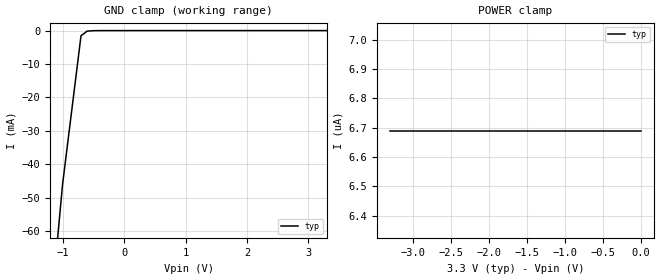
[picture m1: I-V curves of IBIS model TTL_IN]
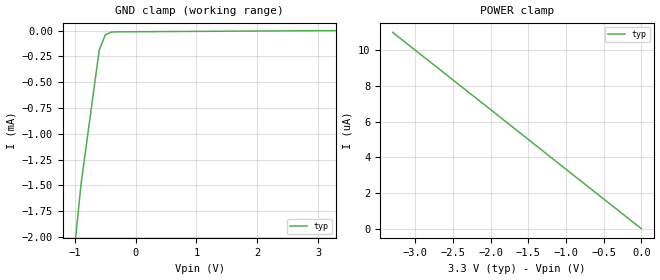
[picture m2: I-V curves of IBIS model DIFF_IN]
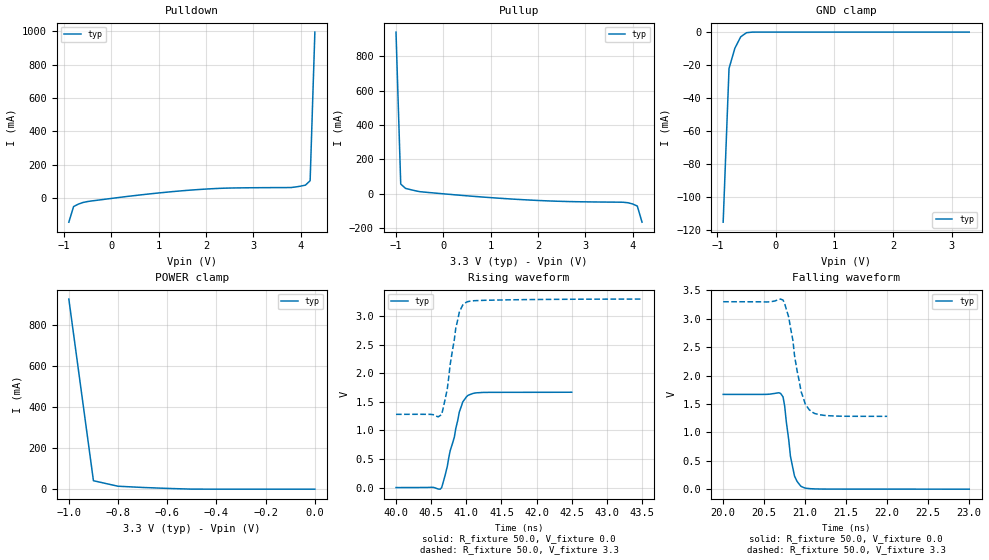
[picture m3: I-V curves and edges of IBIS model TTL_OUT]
|   Texas Instruments Incorporated
|   Data Transmissions Products
|   IBIS Model for SN65LVDS152
|   32DA Package
[IBIS Ver]   3.2
[Comment char]   |_char
[File name]   lvds152.ibs
[File Rev]   1.0
[Date]   11Dec00
[Source]   File originated at Texas Instruments Incorporated.
   Data Transmission Products Group. All data based on
   Bench Measurements.
[Notes]   File created by Thomas Fisher
[Disclaimer]
(C) Copyright Texas Instruments Incorporated 2000
   All rights reserved
  Texas Instruments Incorporated hereby grants the user of this IBIS
model a non-exclusive, nontransferable license to use this IBIS model
under the following terms.  Before using this IBIS model, the user
should read this license.  If the user does not accept these terms,
the IBIS model should be returned to Texas Instruments within 30 days.
  The user is granted this license only to use the IBIS model and
is not granted rights to sell, load, rent, lease or license the IBIS
model in whole or in part, or in modified form to anyone other than
user.  User may modify the IBIS model to suit its specific applications
but rights to derivative works and such modifications shall belong to
Texas Instruments.
  This IBIS model is provided on an "AS IS" basis and Texas Instruments
makes absolutely no warranty with respect to the information contained
herein.  TEXAS INSTRUMENTS DISCLAIMS AND CUSTOMER WAIVES ALL WARRANTIES,
EXPRESS OR IMPLIED, INCLUDING WARRANTIES OF MERCHANTABILITY OR FITNESS
FOR A PARTICULAR PURPOSE. The entire risk as to quality and performance
is with the Customer. ACCORDINGLY, IN NO EVENT SHALL THE COMPANY BE LIABLE
FOR ANY DAMAGES, WHETHER IN CONTRACT OR TORT,INCLUDING ANY LOST PROFITS
OR OTHER INCIDENTAL, CONSEQUENTIAL, EXEMPLARY, OR PUNITIVE DAMAGES ARISING
OUT OF THE USE OR APPLICATION OF THE IBIS model provided in this package.
Further, Texas Instruments reserves the right to discontinue or make changes
without notice to any product herein to improve reliability, function, or
design. Texas Instruments does not convey any license under patent rights
or any other intellectual property rights, including those of third parties.
Contact Texas Instruments at ATTN:DATA TRANSMISSIONS
[Copyright]   Copyright 2000, Texas Instruments, All Rights Reserved
[Component]   SN65LVDS152DA
[Manufacturer]  Texas Instruments Incorporated
[Package]
|   typ   min   max
R_pkg   0.002   0.001   0.003
L_pkg   1.466nH   1.067nH   2.360nH
C_pkg   0.459pF   0.360pF   0.629pF
[Pin] signal_name  model_name   R_pin   L_pin   C_pin
 1   DI+   DIFF_IN   0.003   2.347n   0.610p
 2   DI-   DIFF_IN   0.002   1.869n   0.531p
 3   GND   GND   0.001   1.487n   0.496p
 4   LCI+   DIFF_IN   0.002   1.356n   0.461p
 5   LCI-   DIFF_IN   0.001   1.262n   0.438p
 6   GND   GND   0.001   1.214n   0.410p
 7   CO_EN   TTL_IN   0.001   1.129n   0.381p
 8   VCC   POWER   0.001   1.067n   0.360p
 9   GND   GND   0.001   1.067n   0.360p
10   VCC   POWER   0.001   1.129n   0.381p
11   VCC   POWER   0.001   1.214n   0.410p
12   GND   GND   0.001   1.262n   0.438p
13   GND   GND   0.002   1.356n   0.461p
14   EN   TTL_IN   0.001   1.428n   0.477p
15   CO-   DIFF_OUT   0.002   1.857n   0.532p
16   CO+   DIFF_OUT   0.003   2.340n   0.608p
17   DO-0   TTL_OUT   0.003   2.340n   0.608p
18   DO-1   TTL_OUT   0.002   1.857n   0.532p
19   DO-2   TTL_OUT   0.001   1.430n   0.477p
20   DO-3   TTL_OUT   0.002   1.358n   0.461p
21   DO-4   TTL_OUT   0.001   1.264n   0.438p
22   DO-5   TTL_OUT   0.001   1.216n   0.409p
23   DO-6   TTL_OUT   0.001   1.131n   0.380p
24   DO-7   TTL_OUT   0.001   1.069n   0.360p
25   DO-8   TTL_OUT   0.001   1.069n   0.360p
26   DO-9   TTL_OUT   0.001   1.132n   0.380p
27   DCO   TTL_OUT   0.001   1.217n   0.409p
28   GND   GND   0.001   1.268n   0.437p
29   MCI+   DIFF_IN   0.002   1.383n   0.422p
30   MCI-   DIFF_IN   0.002   1.522n   0.477p
31   LVI   TTL_IN   0.002   1.901n   0.567p
32   VCC   POWER   0.003   2.360n   0.629p
[Diff_pin]   inv_pin   vdiff   tdelay_typ   tdelay_min   tdelay_max
| The 'xx+' pin is diff_pin and the 'xx-' pin is the inv_pin
1   2   100mV   0   0   0
4   5   100mV   0   0   0
29   30   100mV   0   0   0
16   15   NA   0   0   0
| Models and submodels in the file (4): TTL_IN (Input), DIFF_IN (Input), TTL_OUT (3-state), DIFF_OUT (3-state)
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|   TTL Input Model
[Model]   TTL_IN
Model_type   Input
|Signals   CO_EN,EN,LVI
Vinh = 2.0
Vinl = 0.8
|   typ   min   max
C_comp   1.0pF   NA   NA
|   typ   min   max
[Temperature Range]   25.0   NA   NA
[Voltage range]   3.3V   3.0   3.6
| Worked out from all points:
|   GND clamp passes 1 mA (typ) near -0.66 V on its own axis
[GND_clamp]
|   Voltage   I(typ)   I(min)   I(max)
-3.3V     -528mA     NA         NA
-1.3V     -106mA     NA         NA
-1V       -46mA      NA         NA
-700mV    -1.54mA    NA         NA
-600mV    -160uA     NA         NA
3.3V      3.69uA     NA         NA
[Power_clamp]
| Note that the[POWER_clamp]voltage table is referenced to Vcc
| and is calculated using Vtable=Vcc - Vmeasured.
|   Voltage   I(typ)   I(min)   I(max)
-3.3V     6.69uA     NA         NA
-2.7V     6.69uA     NA         NA
-2V       6.69uA     NA         NA
-800mV    6.69uA     NA         NA
0V        6.69uA     NA         NA
|   Differential Input Model
[Model]   DIFF_IN
Model_type   Input
|Signals   DI+,DI-,LCI+,LCI-,MCI+,MCI-
Vinh = 2.0
Vinl = 0.8
|   typ   min   max
C_comp   1.0pF   NA   NA
|   typ   min   max
[Temperature Range]   25.0   NA   NA
[Voltage range]   3.3V   3.0   3.6
[GND_clamp]
|   Voltage   I(typ)   I(min)   I(max)
-3.3V     -19.6mA    NA         NA
-1.2V     -3.25mA    NA         NA
-900mV    -1.49mA    NA         NA
-600mV    -188uA     NA         NA
-500mV    -42.1uA    NA         NA
-400mV    -14.3uA    NA         NA
-300mV    -12.1uA    NA         NA
3.3V      125pA      NA         NA
[Power_clamp]
| Note that the[POWER_clamp]voltage table is referenced to Vcc
| and is calculated using Vtable=Vcc - Vmeasured.
|   Voltage   I(typ)   I(min)   I(max)
-3.3V     11uA       NA         NA
-3V       10uA       NA         NA
-2V       6.67uA     NA         NA
-1V       3.33uA     NA         NA
0V        125pA      NA         NA
|   Parallel Data & Data Clock Output Model
[Model]   TTL_OUT
Model_type   3-state
|Signals   DI-0,DI-1,DI-2,DI-3,DI-4,DI-5,DI-6,DI-7,DI-8,DI-9.DCO
Vmeas = 1.5V   |Reference voltage for timing measurements
Cref = 8pF   |Timing specification test load capacitance value
Vref = 0   |Timing specification test load voltage; GND
| variable   typ   min   max
C_comp   1.0pF   NA   NA
|   typ   min   max
[Temperature Range]   25.0   NA   NA
[Voltage range]   3.3V   3.0V   3.6V
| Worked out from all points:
|   slope of the pulldown table from 0 to 0.495 V, typ, clamps not added: 28.9 ohm
|   slope of the pullup table from 0 to 0.495 V, typ, clamps not added: 42.7 ohm
|   GND clamp passes 1 mA (typ) near -0.53 V on its own axis
|   POWER clamp passes 1 mA (typ) near -0.52 V on its own axis
|   rising waveform, R_fixture 50.0, V_fixture 0.0: 20-80 % time 182ps typ, NA min, NA max; typ from 0 V to 1.67 V
|   falling waveform, R_fixture 50.0, V_fixture 0.0: 20-80 % time 96ps typ, NA min, NA max; typ from 1.67 V to 0 V
|   rising waveform, R_fixture 50.0, V_fixture 3.3: 20-80 % time 148ps typ, NA min, NA max; typ from 1.28 V to 3.3 V
|   falling waveform, R_fixture 50.0, V_fixture 3.3: 20-80 % time 143ps typ, NA min, NA max; typ from 3.3 V to 1.28 V
[Pulldown]
|   Voltage   I(typ)   I(min)   I(max)
-900mV    -142mA     NA         NA
-800mV    -48.8mA    NA         NA
-700mV    -34.1mA    NA         NA
-500mV    -18.3mA    NA         NA
600mV     20.6mA     NA         NA
1.7V      50.3mA     NA         NA
2.4V      61.3mA     NA         NA
3.8V      65.2mA     NA         NA
4.1V      79.4mA     NA         NA
4.2V      106mA      NA         NA
4.3V      994mA      NA         NA
[Pullup]
|   Voltage   I(typ)   I(min)   I(max)
| Note that the[Pullup]voltage table is referenced to Vcc
| and is calculated using Vtable=Vcc - Vmeasured.
-1V       940mA      NA         NA
-900mV    56.8mA     NA         NA
-800mV    31.7mA     NA         NA
-500mV    12.5mA     NA         NA
1.4V      -29.6mA    NA         NA
2.4V      -43.1mA    NA         NA
3.9V      -51.8mA    NA         NA
4.1V      -71.3mA    NA         NA
4.2V      -165mA     NA         NA
[GND_clamp]
|   Voltage   I(typ)   I(min)   I(max)
| Outputs in High Impedance (off)
-900mV    -115mA     NA         NA
-800mV    -22mA      NA         NA
-700mV    -9.74mA    NA         NA
-600mV    -2.83mA    NA         NA
-500mV    -348uA     NA         NA
-400mV    -20.7uA    NA         NA
-300mV    -762nA     NA         NA
-200mV    -21.4nA    NA         NA
-100mV    -533pA     NA         NA
0V        -21.7pA    NA         NA
3.3V      242pA      NA         NA
[POWER_clamp]
|   Voltage   I(typ)   I(min)   I(max)
| Note that the [POWER_clamp] voltage table is referenced to Vcc
| and is calculated using Vtable = Vcc - Vmeasured.
| Outputs in Tri-state.
-1V       928mA      NA         NA
-900mV    41.2mA     NA         NA
-800mV    14.3mA     NA         NA
-700mV    8.37mA     NA         NA
-600mV    3.7mA      NA         NA
-500mV    196uA      NA         NA
-400mV    22.3uA     NA         NA
-300mV    1.24uA     NA         NA
-200mV    44.4nA     NA         NA
-100mV    1.4nA      NA         NA
0V        242pA      NA         NA
[Ramp]
|   typ   min   max
dV/dt_r   1.00V/190ps   NA   NA
dV/dt_f   1.21V/170ps   NA   NA
R_load = 50
[Rising Waveform]
R_fixture = 50.0
V_fixture = 0.0
C_fixture = 0p
L_fixture = 0n
|   V(typ)   V(min)   V(max)
40ns      0V         NA         NA
40.65ns   1mV        NA         NA
40.73ns   372mV      NA         NA
40.77ns   642mV      NA         NA
40.83ns   882mV      NA         NA
40.9ns    1.32V      NA         NA
40.95ns   1.499V     NA         NA
41.02ns   1.61V      NA         NA
41.25ns   1.665V     NA         NA
42.5ns    1.668V     NA         NA
[Falling Waveform]
R_fixture = 50.0
V_fixture = 0.0
C_fixture = 0p
L_fixture = 0n
|   V(typ)   V(min)   V(max)
20ns      1.669V     NA         NA
20.7ns    1.686V     NA         NA
20.73ns   1.625V     NA         NA
20.75ns   1.463V     NA         NA
20.8ns    863mV      NA         NA
20.82ns   583mV      NA         NA
20.87ns   231mV      NA         NA
20.93ns   82mV       NA         NA
20.98ns   30mV       NA         NA
23ns      0V         NA         NA
[Rising Waveform]
R_fixture = 50.0
V_fixture = 3.3
C_fixture = 0p
L_fixture = 0n
|   V(typ)   V(min)   V(max)
40ns      1.281V     NA         NA
40.6ns    1.237V     NA         NA
40.65ns   1.278V     NA         NA
40.73ns   1.728V     NA         NA
40.77ns   2.148V     NA         NA
40.85ns   2.784V     NA         NA
40.9ns    3.066V     NA         NA
40.95ns   3.195V     NA         NA
41ns      3.243V     NA         NA
43.5ns    3.298V     NA         NA
[Falling Waveform]
R_fixture = 50.0
V_fixture = 3.3
C_fixture = 0p
L_fixture = 0n
|   V(typ)   V(min)   V(max)
20ns      3.3V       NA         NA
20.73ns   3.329V     NA         NA
20.8ns    3.026V     NA         NA
20.85ns   2.622V     NA         NA
20.87ns   2.354V     NA         NA
20.95ns   1.718V     NA         NA
21ns      1.502V     NA         NA
21.1ns    1.344V     NA         NA
21.35ns   1.288V     NA         NA
22ns      1.282V     NA         NA
